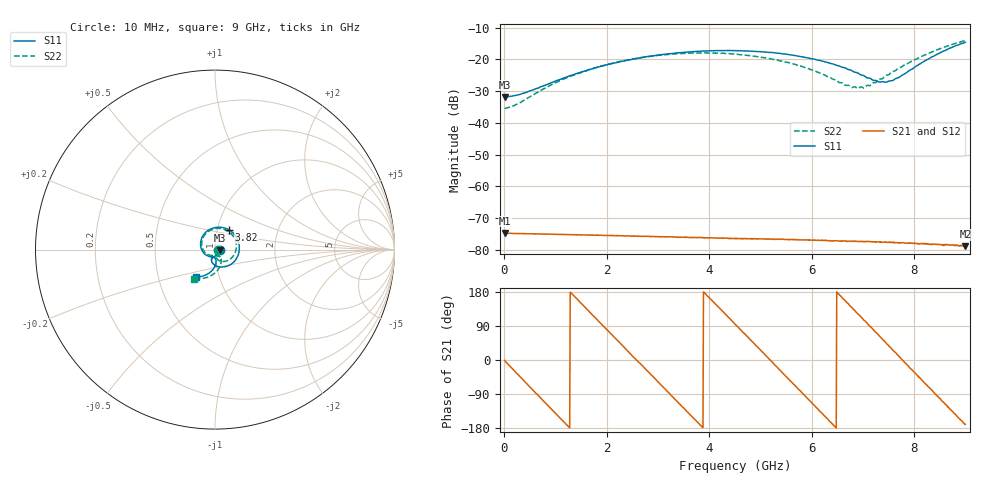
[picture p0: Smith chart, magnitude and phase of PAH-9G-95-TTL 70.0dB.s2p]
! MTS Systemtechnik GmbH
! S-Parameters
! Model: PAH-9G/95-TTL
! Attenuation Step: 70.0dB
#  HZ  S  DB  R  50.00
! Rohde & Schwarz Vector Network Analyzer
! Rohde-Schwarz,ZNB20-2Port,1334333062101652,3.45
! Created: UTC 1/26/2024, 7:23:38 AM
! freq[Hz]  db:S11  ang:S11  db:S21  ang:S21  db:S12  ang:S12  db:S22  ang:S22
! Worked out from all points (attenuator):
!   900 points, 10 MHz to 9 GHz, reference 50 ohm
!   highest |S21| = -74.70 dB at 10 MHz (marker M1); lowest = -78.9 dB at 9 GHz (marker M2)
!   lowest |S11| = -31.9 dB at 20 MHz (marker M3), VSWR 1.05, Z = 52.6 - j0.248 ohm
!   |S11| at or under -10 dB: start of sweep to end of sweep
!   |S22| runs from -35.4 to -14.0 dB; largest |S21 - S12| = 7.9e-06
!   S11 on the Smith chart (normalised r, x): 10 MHz: 1.05, -0.01; 3.82 GHz: 1.14, +0.25; 9 GHz: 0.77, -0.24
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1e7  -31.80 -5.9  -74.70 -0.9  -74.71 -1.4  -35.37 -8.7
2e7  -31.85 -5.3  -74.81 -2.7  -74.83 -2.9  -35.44 -7.3
1.6e8  -31.56 -22.8  -74.85 -22.8  -74.86 -22.6  -34.84 -30.1
4.1e8  -30.53 -54.9  -74.93 -58.1  -74.99 -57.9  -32.75 -68.4
9.6e8  -27.13 -113.4  -75.14 -134.8  -75.19 -135.1  -27.71 -128.4
1.51e9  -23.94 -158.3  -75.40 148.8  -75.38 148.8  -24.07 -172.3
2.14e9  -21.20 157.6  -75.59 61.4  -75.60 61.0  -21.09 145.1
3.01e9  -18.64 103.2  -75.84 -58.4  -75.94 -58.3  -18.73 92.4
3.82e9  -17.46 54.9  -76.16 -170.9  -76.22 -170.6  -17.99 46.7
4.51e9  -17.26 14.6  -76.37 94.0  -76.44 94.7  -18.35 8.7
5.31e9  -18.03 -32.5  -76.69 -16.3  -76.67 -15.6  -20.14 -34.6
6.01e9  -19.83 -72.5  -76.92 -114.4  -77.02 -112.7  -23.33 -67.8
6.66e9  -22.76 -102.8  -77.26 155.7  -77.34 156.7  -28.18 -79.7
6.9e9  -24.29 -109.1  -77.36 122.0  -77.42 123.2  -29.17 -71.0
7.02e9  -25.15 -109.9  -77.43 104.9  -77.47 106.9  -29.00 -64.9
7.14e9  -25.99 -109.2  -77.44 89.2  -77.57 89.6  -28.25 -59.6
7.32e9  -27.13 -103.4  -77.56 63.6  -77.66 64.7  -26.29 -55.7
7.51e9  -26.83 -94.6  -77.68 36.2  -77.74 37.8  -24.75 -56.7
7.71e9  -25.63 -86.9  -77.86 8.1  -77.79 10.3  -22.68 -61.1
8.21e9  -20.47 -90.5  -78.20 -61.7  -78.30 -59.0  -18.59 -83.2
8.66e9  -16.73 -108.3  -78.52 -124.8  -78.51 -121.1  -15.76 -107.0
9e9  -14.59 -125.1  -78.88 -170.0  -78.66 -168.9  -14.04 -125.7
